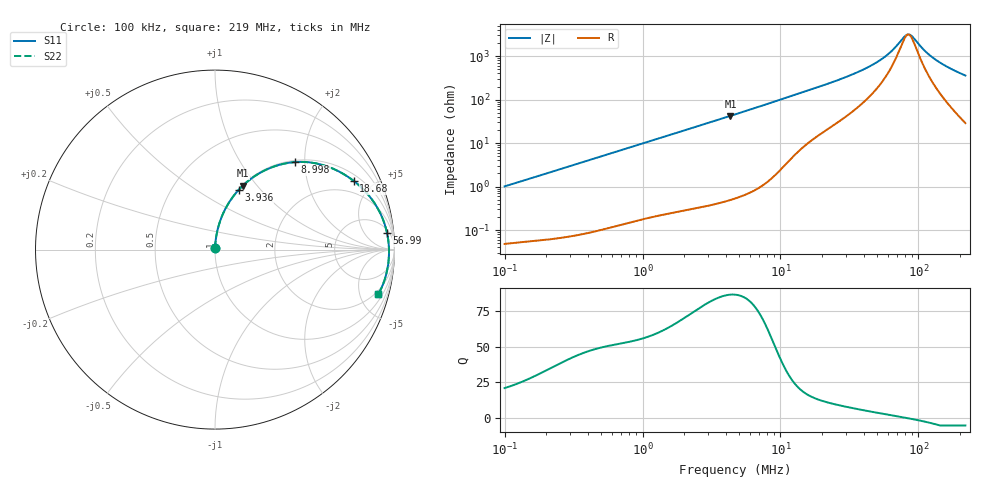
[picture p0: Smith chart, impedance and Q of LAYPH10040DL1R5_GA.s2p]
! LAYPH10040DL1R5_GA  S-PARAMETER MODEL  ( General Type )
! Model Generated by TAIYO YUDEN Corporation (http://www.ty-top.com)
! Version 1.0
! TAIYO YUDEN Control No. 180920NI43SB-FBB
! Copyright(c) 2018 TAIYO YUDEN CO.,LTD. All Rights Reserved.
! Product Description (link to TY-COMPAS)
! https://ds.yuden.co.jp/TYCOMPAS/or/detail?pn=LAYPH10040DL1R5NGA&u=M
! Products Name : Inductors
! Characteristics :
!  Inductance : 1.5 uH , SRF(min) : -Hz , DC Resistance(max) : 0.012 Ohm
!  Rated Current : Saturation :8.6 A , Temp Rise : 3.3 A (25 degC)
!  Case Size : 10.1 x 10.0 / 0.398 x 0.394 [mm/inch] , Thickness : 4 / 0.157 [mm/inch]
!  (Conditions: Temperature = 25 degC , DC Bias Current/Voltage = 0A / 0V)
! External Node Assignments :
!  1  o---GGG---o  2
! GND o---------o GND
! Frequency Range : 0.1MHz  -  218.972167MHz  [ 402 STEP ]
# MHz S RI R 50
! Freq[MHz].  S11 Real  S11 Imag  S21 Real  S21 Imag  S12 Real  S12 Imag  S22 Real  S22 Imag
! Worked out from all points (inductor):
!   401 points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, 100 kHz to 219 MHz, reference 50 ohm
!   read as one part in series: L = 1.6 uH near 103.9 kHz
!   highest Q = 86.2 at 4.333 MHz (marker M1), where L = 1.55 uH
!   self-resonance near 84.32 MHz
!   S11 on the Smith chart (normalised r, x): 100 kHz: 1.00, +0.02; 3.936 MHz: 1.01, +0.77; 8.998 MHz: 1.03, +1.80; 18.68 MHz: 1.29, +3.87; 56.99 MHz: 7, +18; 219 MHz: 1.58, -7.15
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0.1  0.00058 0.0101  0.9994 -0.0101  0.9994 -0.0101  0.00058 0.0101
0.362673  0.00208 0.0359  0.9979 -0.0359  0.9979 -0.0359  0.00208 0.0359
1.315317  0.0183 0.1261  0.9817 -0.1261  0.9817 -0.1261  0.0183 0.1261
2.433668  0.056 0.2233  0.944 -0.2233  0.944 -0.2233  0.056 0.2233
3.935824  0.1315 0.3321  0.8685 -0.3321  0.8685 -0.3321  0.1315 0.3321
4.333019  0.1548 0.3559  0.8452 -0.3559  0.8452 -0.3559  0.1548 0.3559
4.770297  0.1815 0.3797  0.8185 -0.3797  0.8185 -0.3797  0.1815 0.3797
8.997617  0.4473 0.4876  0.5527 -0.4876  0.5527 -0.4876  0.4473 0.4876
12.00583  0.5941 0.473  0.4059 -0.473  0.4059 -0.473  0.5941 0.473
16.97108  0.7404 0.4059  0.2596 -0.4059  0.2596 -0.4059  0.7404 0.4059
18.68377  0.7733 0.3824  0.2267 -0.3824  0.2267 -0.3824  0.7733 0.3824
36.62254  0.9212 0.2016  0.0788 -0.2016  0.0788 -0.2016  0.9212 0.2016
47.02309  0.9466 0.1376  0.0534 -0.1376  0.0534 -0.1376  0.9466 0.1376
56.99291  0.9588 0.0909  0.0412 -0.0909  0.0412 -0.0909  0.9588 0.0909
61.54953  0.9623 0.0728  0.0377 -0.0728  0.0377 -0.0728  0.9623 0.0728
79.02916  0.9688 0.0149  0.0312 -0.0149  0.0312 -0.0149  0.9688 0.0149
85.34759  0.9695 -0.00281  0.0305 0.00281  0.0305 0.00281  0.9695 -0.00281
90.41577  0.9695 -0.0161  0.0305 0.0161  0.0305 0.0161  0.9695 -0.0161
111.7133  0.9667 -0.066  0.0333 0.066  0.0333 0.066  0.9667 -0.066
132.82  0.9604 -0.1087  0.0396 0.1087  0.0396 0.1087  0.9604 -0.1087
167.292  0.9445 -0.1697  0.0555 0.1697  0.0555 0.1697  0.9445 -0.1697
218.9722  0.9109 -0.2475  0.0891 0.2475  0.0891 0.2475  0.9109 -0.2475
